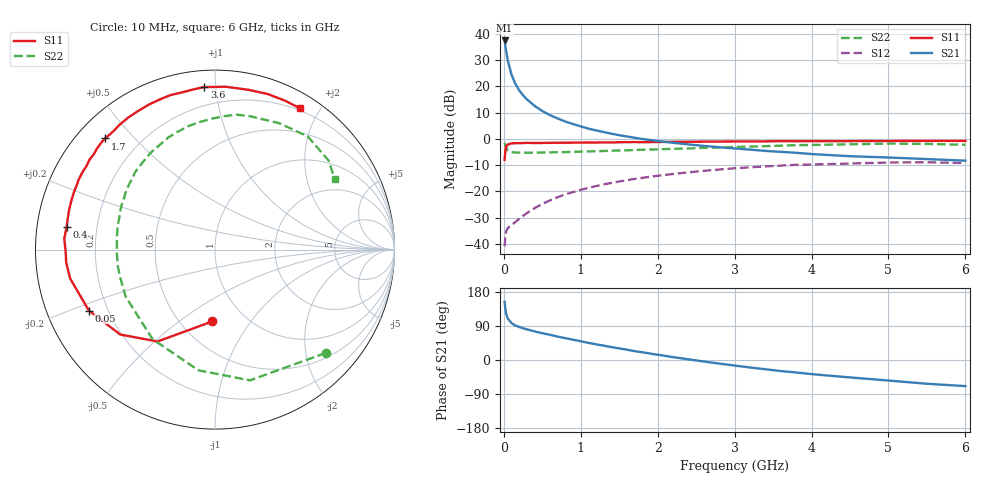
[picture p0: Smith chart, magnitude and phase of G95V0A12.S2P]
! SIEMENS Small Signal Semiconductors
! BFG235
! Si NPN RF Bipolar Junction Transistor in SOT223
! VCE = 5 V  IC = 120 mA
! Common Emitter S-Parameters:  July  1994
# GHz  S  MA  R  50
!  f  S11  S21  S12  S22
! GHz  MAG  ANG  MAG  ANG  MAG  ANG  MAG  ANG
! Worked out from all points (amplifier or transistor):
!   40 points, 10 MHz to 6 GHz, reference 50 ohm
!   highest |S21| = 37.5 dB at 10 MHz (marker M1)
!   |S21| within 3 dB of that: start of sweep to 24.89 MHz
!   unconditionally stable (mu >= 1): 453.3 MHz to 1.465 GHz
!   at 200 MHz: K = 0.79, MSG = 24.4 dB, |S12| = -30.4 dB
!   at 1.5 GHz: K = 0.99, MSG = 8.8 dB, |S12| = -16.2 dB
!   at 6 GHz: K = 0.90, MSG = 0.4 dB, |S12| = -9.1 dB
!   S11 on the Smith chart (normalised r, x): 10 MHz: 0.71, -0.67; 50 MHz: 0.13, -0.23; 400 MHz: 0.09, +0.08; 1.7 GHz: 0.08, +0.41; 3.6 GHz: 0.09, +0.93; 6 GHz: 0.17, +1.75
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0.01  0.4004 -92.1  74.92 153.3  0.0091 63.5  0.8442 -43.0
0.02  0.6035 -122.0  59.47 134.6  0.0145 50.7  0.7541 -75.0
0.03  0.7088 -138.1  47.06 122.7  0.0174 42.3  0.6788 -97.8
0.05  0.7805 -154.2  31.53 109.8  0.0201 34.3  0.6082 -124.9
0.1  0.8229 -168.7  16.72 97.3  0.023 35.3  0.5627 -152.2
0.15  0.8325 -175.2  11.24 91.1  0.0262 42.1  0.5505 -163.6
0.2  0.8315 -178.7  8.411 87.1  0.0303 46.6  0.5495 -170.0
0.25  0.8363 178.2  6.775 83.6  0.0343 50.1  0.5468 -174.4
0.3  0.842 175.9  5.66 80.9  0.0388 53.1  0.5473 -178.1
0.4  0.8366 171.3  4.255 75.4  0.0483 56.3  0.5471 176.8
0.5  0.8386 167.7  3.401 70.6  0.0579 57.4  0.5513 172.5
0.6  0.8429 164.7  2.837 66.5  0.0678 57.4  0.5547 168.7
0.7  0.8453 161.1  2.447 61.8  0.0779 57.2  0.559 165.2
0.9  0.8495 155.6  1.919 53.5  0.0974 54.6  0.5672 159.0
1.1  0.8553 149.3  1.571 45.1  0.1172 51.5  0.5792 152.9
1.7  0.8713 134.7  1.054 23.4  0.1734 39.4  0.6173 136.7
2.2  0.8804 123.4  0.844 7.6  0.2153 28.5  0.6487 123.2
3.2  0.895 102.0  0.626 -19.7  0.2886 5.3  0.7153 97.1
3.6  0.9078 93.8  0.568 -29.2  0.3111 -4.6  0.7452 86.0
4.5  0.9095 78.2  0.469 -46.0  0.3405 -24.5  0.7898 63.1
5.5  0.9168 64.9  0.414 -62.7  0.3592 -46.5  0.8042 37.9
6  0.9186 59.0  0.386 -68.9  0.349 -54.8  0.773 30.4
